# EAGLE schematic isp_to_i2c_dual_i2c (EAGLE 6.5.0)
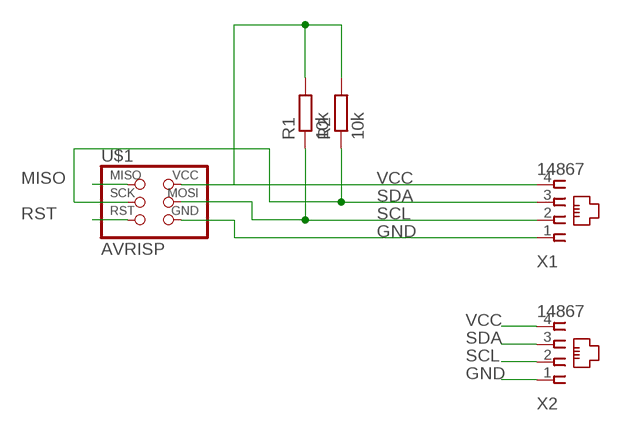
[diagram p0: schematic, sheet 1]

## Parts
R1  10k  R-EU_M1206  [M1206]
R2  10k  R-EU_M1206  [M1206]
U$1  AVRISP  [2X03]
X1  14867  [14867]
X2  14867  [14867]

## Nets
GND: U$1.6(GND) X1.1 X2.1
MISO: U$1.1(MISO)
RST: U$1.5(RST)
SCL: R1.1 U$1.4(MOSI) X1.2 X2.2
SDA: R2.1 U$1.3(SCK) X1.3 X2.3
VCC: R1.2 R2.2 U$1.2(VCC) X1.4 X2.4

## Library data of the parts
R1 R2 = resistor:R-EU_: RESISTOR, European symbol
U$1 = fab:AVRISP
X1 X2 = con-4ucon:14867: RJ11 Connector Source: 4UCON TECHNOLOGY INC. 14867.pdf; OC_FARNELL: unknown; OC_NEWARK: unknown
